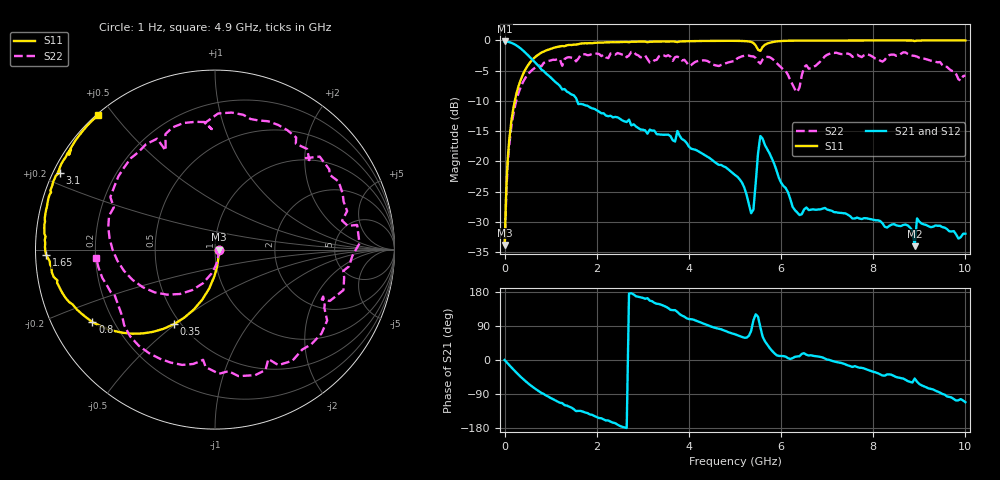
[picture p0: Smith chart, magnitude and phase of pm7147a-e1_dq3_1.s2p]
# GHz S DB R 50
! S-Parameters data
! Freq  dbS11  angS11  dbS21  angS21  dbS12  angS12  dbS22  angS22
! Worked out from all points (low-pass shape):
!   279 points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, 1 Hz to 10 GHz, reference 50 ohm
!   highest |S21| = -0.18 dB at 1.6 Hz (marker M1); lowest = -34.0 dB at 8.9 GHz (marker M2)
!   |S21| within 3 dB of the highest: start of sweep to 602.3 MHz
!   lowest |S11| = -33.8 dB at 631 Hz (marker M3), VSWR 1.04, Z = 52.1 - j6.78e-05 ohm
!   |S11| at or under -10 dB: start of sweep to 221.9 MHz
!   |S22| runs from -33.8 to -1.9 dB; largest |S21 - S12| = 1.7e-12
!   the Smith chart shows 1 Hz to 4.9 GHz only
!   S11 on the Smith chart (normalised r, x): 1 Hz: 1.04, -0.00; 350 MHz: 0.46, -0.49; 800 MHz: 0.12, -0.27; 1.65 GHz: 0.03, -0.02; 3.1 GHz: 0.02, +0.23; 4.9 GHz: 0.00, +0.46
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1e-09  -33.85 -0.0  -0.18 -0.0  -0.18 -0.0  -33.85 -0.0
1.6e-09  -33.85 -0.0  -0.18 -0.0  -0.18 -0.0  -33.85 -0.0
6.31e-07  -33.85 -0.0  -0.18 -0.0  -0.18 -0.0  -33.85 -0.0
0.1  -16.51 -91.4  -0.28 -13.3  -0.28 -13.3  -17.39 -98.3
0.35  -6.50 -118.8  -1.34 -44.5  -1.34 -44.5  -7.70 -144.7
0.8  -2.00 -149.4  -4.83 -86.9  -4.83 -86.9  -4.28 157.4
1.65  -0.53 -178.3  -10.51 -134.3  -10.51 -134.3  -2.40 88.7
1.7  -0.49 -179.7  -10.57 -136.3  -10.57 -136.3  -2.28 83.1
2.5  -0.27 164.2  -12.94 -173.8  -12.94 -173.8  -2.20 23.6
3.1  -0.30 153.6  -15.43 163.1  -15.43 163.1  -3.09 -24.1
3.35  -0.18 151.1  -15.53 147.8  -15.53 147.8  -2.62 -32.3
4.15  -0.11 140.7  -18.11 104.0  -18.11 104.0  -3.51 -105.9
4.9  -0.06 130.9  -21.61 71.5  -21.61 71.5  -3.56 -175.8
5.05  -0.07 128.8  -22.54 65.6  -22.54 65.6  -2.95 171.9
5.4  -0.43 121.2  -27.97 104.9  -27.97 104.9  -2.64 133.9
5.55  -1.73 127.2  -15.81 86.7  -15.81 86.7  -3.84 124.9
6.1  -0.07 121.7  -24.42 8.8  -24.42 8.8  -5.06 80.8
6.7  -0.02 115.1  -27.94 10.9  -27.94 10.9  -4.36 79.7
7.45  -0.01 108.2  -28.83 -14.2  -28.83 -14.2  -2.19 35.8
8.35  -0.01 101.0  -30.66 -37.9  -30.66 -37.9  -2.41 -3.8
8.9  -0.12 96.1  -34.03 -48.8  -34.03 -48.8  -2.57 -40.1
10  -0.01 89.9  -31.97 -111.4  -31.97 -111.4  -5.80 -111.5
